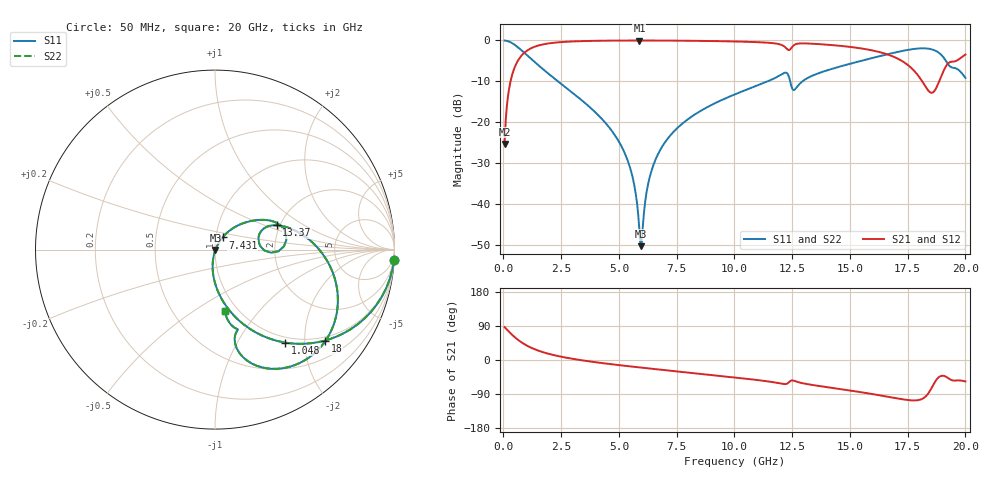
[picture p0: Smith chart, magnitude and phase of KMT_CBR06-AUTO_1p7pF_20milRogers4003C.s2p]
! Data measured by Modelithics Inc. support@modelithics.com 813-866-6335
! KEMET CBR06-AUTO 1.7pF, Pad Width= 0.851mm, Pad Length= 0.64mm, Pad Gap= 0.62mm, 20mil Rogers 4003C substrate Data, January 2022
# hz S ma R 50
! 2 Port Network Data from SP1.SP block
! freq  magS11  angS11  magS21  angS21  magS12  angS12  magS22  angS22
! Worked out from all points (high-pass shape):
!   401 points, 50 MHz to 20 GHz, reference 50 ohm
!   highest |S21| = -0.03 dB at 5.885 GHz (marker M1); lowest = -25.3 dB at 50 MHz (marker M2)
!   |S21| within 3 dB of the highest: 900.9 MHz to 16.39 GHz (15.49 GHz wide, 179 % of centre)
!   lowest |S11| = -50.3 dB at 5.935 GHz (marker M3), VSWR 1.01, Z = 50.2 - j0.202 ohm
!   |S11| at or under -10 dB: 2.36 GHz to 11.44 GHz (9.079 GHz wide, 132 % of centre); 12.41 GHz to 12.95 GHz (531.7 MHz wide, 4.19 % of centre)
!   |S22| runs from -50.3 to 0.0 dB; largest |S21 - S12| = 0
!   S11 on the Smith chart (normalised r, x): 50 MHz: 1, -35; 1.048 GHz: 0.91, -1.62; 7.431 GHz: 1.08, +0.15; 13.37 GHz: 1.92, +0.60; 18 GHz: 0.89, -2.49; 20 GHz: 0.87, -0.68
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5e7  0.9985 -3.3  0.05418 86.7  0.05418 86.7  0.9985 -3.3
2.495e8  0.965 -16.0  0.2617 73.9  0.2617 73.9  0.965 -16.0
3.99125e8  0.9167 -24.8  0.3987 65.1  0.3987 65.1  0.9167 -24.8
1.0475e9  0.6491 -52.9  0.7592 36.9  0.7592 36.9  0.6491 -52.9
1.94525e9  0.3924 -73.2  0.9178 16.5  0.9178 16.5  0.3924 -73.2
3.391625e9  0.1856 -90.0  0.9802 -0.8  0.9802 -0.8  0.1856 -90.0
5.237e9  0.04284 -101.6  0.9962 -15.2  0.9962 -15.2  0.04284 -101.6
5.636e9  0.01871 -99.3  0.9968 -17.9  0.9968 -17.9  0.01871 -99.3
5.885375e9  0.00488 -73.8  0.9969 -19.6  0.9969 -19.6  0.00488 -73.8
5.93525e9  0.003068 -41.0  0.9969 -19.9  0.9969 -19.9  0.003068 -41.0
6.33425e9  0.02148 59.6  0.9966 -22.5  0.9966 -22.5  0.02148 59.6
6.73325e9  0.04307 60.9  0.9958 -25.1  0.9958 -25.1  0.04307 60.9
7.4315e9  0.07995 58.2  0.9933 -29.5  0.9933 -29.5  0.07995 58.2
1.0025e10  0.2196 42.6  0.9703 -46.1  0.9703 -46.1  0.2196 42.6
1.216962e10  0.4022 15.0  0.8388 -63.5  0.8388 -63.5  0.4022 15.0
1.2419e10  0.3122 -3.2  0.7774 -55.4  0.7774 -55.4  0.3122 -3.2
1.336662e10  0.3699 21.5  0.9115 -65.8  0.9115 -65.8  0.3699 21.5
1.670825e10  0.6857 -13.5  0.6614 -97.7  0.6614 -97.7  0.6857 -13.5
1.8005e10  0.7983 -39.7  0.3558 -105.3  0.3558 -105.3  0.7983 -39.7
1.86035e10  0.7683 -58.8  0.2325 -66.2  0.2325 -66.2  0.7683 -58.8
1.915212e10  0.5643 -77.6  0.4793 -44.0  0.4793 -44.0  0.5643 -77.6
2e10  0.3482 -80.8  0.6717 -56.5  0.6717 -56.5  0.3482 -80.8
